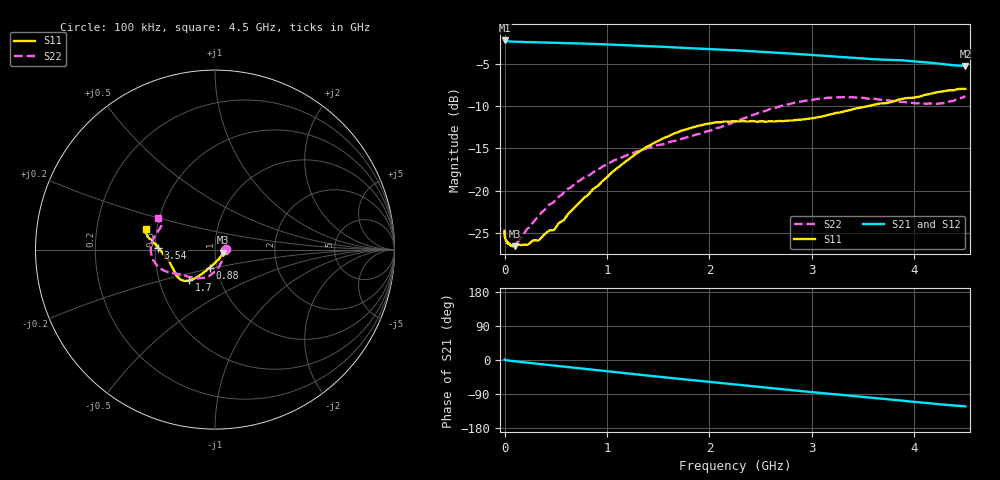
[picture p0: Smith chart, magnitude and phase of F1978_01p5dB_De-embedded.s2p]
! Integrated Device Technology
! Corporate Headquarters
! 6024 Silver Creek Valley Road
! San Jose, CA 95138  USA
! Phone:  1-408-284-8200
! Toll Free:  1-800-223-1366
! Webpage:  http://www.idt.com/
! Timing and RF Division
! 515 Groton Road, Suite 102
! Westford, MA 01886-6024
! Device:  F1978
! Description: 6-bit, 75 ohm, 0.5 dB Digital Step Attenuator
! Frequency:  5.0 MHz -  3.00 GHz
! Package:  4x4 mm QFN Plastic Package: 20 pin
! Ports:  2 RF, 11 DC
!  Pin  1  = D5 (16 dB)
!  Pin  2  = RF1  =  Port 1
!  Pin  3  = Serial Data In (DATA)
!  Pin  4  = Serial Clock (CLK)
!  Pin  5  = Serial Latch Enable (LE)
!  Pin  6  = VDD
!  Pin  7  = NC
!  Pin  8  = NC
!  Pin  9  = NC
!  Pin 10  = GND
!  Pin 11  = GND
!  Pin 12  = NC
!  Pin 13  = VMODE
!  Pin 14  = RF2  =  Port 2
!  Pin 15  = D4 (8 dB)
!  Pin 16  = D3 (4 dB)
!  Pin 17  = D2 (2 dB)
!  Pin 18  = NC
!  Pin 19  = D1 (1 dB)
!  Pin 20  = D0 (0.5 dB)
! State:  3
! Atten State:  1.5 dB
! Voltage:  +3.30 Volts
! Current:  0.565 mA
! Data:  The device was measured on a F1975 evaluation board which has
!  individual transmission lines to the RF pins.  Data was collected
!  using a calibrated network analyzer.  The evaluation board was
!  de-embedded using Automatic Fixture Removal (AFR).
!  The reference plane is the edge of the package pin.
! Misc:
!  Action Tracker AT0416
! Date Measured:  2018-02-08
! Date:  2018-03-26  MJV
! Note:
!  Integrated Device Technology supplies this data as a sample of measured
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# GHz S dB R 75
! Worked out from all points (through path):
!   291 points, 100 kHz to 4.5 GHz, reference 75 ohm
!   highest |S21| = -2.19 dB at 100 kHz (marker M1); lowest = -5.2 dB at 4.5 GHz (marker M2)
!   group delay of S21, straight-line fit = 76.6 ps
!   lowest |S11| = -26.6 dB at 100 MHz (marker M3), VSWR 1.10, Z = 81.8 - j2.68 ohm
!   |S11| at or under -10 dB: start of sweep to 3.541 GHz
!   |S22| runs from -26.6 to -8.8 dB; largest |S21 - S12| = 0.00021
!   S11 on the Smith chart (normalised r, x): 100 kHz: 1.12, +0.00; 880 MHz: 0.93, -0.19; 1.7 GHz: 0.71, -0.26; 3.54 GHz: 0.52, +0.01; 4.5 GHz: 0.43, +0.12
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0.0001  -24.84 0.4  -2.19 1.2  -2.20 1.2  -24.60 0.9
0.0008  -25.33 -1.4  -2.23 1.0  -2.23 1.0  -25.06 -0.6
0.003  -25.55 -1.7  -2.25 0.7  -2.25 0.7  -25.37 -1.1
0.02  -26.06 -6.2  -2.28 -0.9  -2.28 -0.9  -25.98 -7.3
0.1  -26.58 -20.4  -2.34 -3.3  -2.34 -3.3  -26.47 -25.4
0.32  -25.93 -52.6  -2.42 -9.9  -2.42 -9.9  -23.14 -56.9
0.44  -24.71 -67.6  -2.45 -13.4  -2.45 -13.4  -21.62 -65.9
0.48  -24.68 -73.1  -2.47 -14.6  -2.47 -14.6  -21.37 -69.5
0.76  -21.06 -99.2  -2.56 -22.8  -2.56 -22.8  -18.59 -87.0
0.88  -19.68 -105.6  -2.61 -26.3  -2.61 -26.3  -17.71 -93.6
1.3  -15.48 -120.6  -2.81 -38.4  -2.81 -38.4  -15.33 -112.6
1.52  -13.99 -125.7  -2.93 -44.6  -2.93 -44.6  -14.56 -121.6
1.7  -13.03 -129.8  -3.05 -49.6  -3.04 -49.6  -13.96 -129.4
1.98  -12.07 -136.1  -3.21 -57.2  -3.21 -57.2  -12.96 -140.1
2.26  -11.77 -144.1  -3.37 -64.8  -3.36 -64.8  -11.78 -148.5
2.68  -11.74 -158.5  -3.66 -76.3  -3.66 -76.3  -10.03 -159.2
3.02  -11.40 -169.4  -3.93 -85.3  -3.93 -85.3  -9.21 -169.5
3.3  -10.66 -176.7  -4.18 -92.5  -4.18 -92.5  -8.92 -179.5
3.54  -10.00 178.3  -4.36 -98.5  -4.36 -98.5  -9.09 173.0
3.76  -9.55 174.7  -4.49 -103.8  -4.49 -103.8  -9.33 166.4
4.22  -8.34 169.0  -4.90 -116.1  -4.90 -116.1  -9.71 155.3
4.5  -7.94 163.7  -5.21 -122.3  -5.21 -122.3  -8.80 151.3
